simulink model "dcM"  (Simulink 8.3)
settings: Solver=ode45  StartTime=0.0  StopTime=2  FixedStep=1e-6  MaxStep=0.00001  RelTol=1e-3  AbsTol=1e-3
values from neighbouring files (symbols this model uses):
  ke = 2    [set_ga.m]
  Ra = Pcun/(Ian^2)    [Ex5i_dcMd.m]    (also in Ex6i_dcMs.m = Pcun/(In^2))
undefined symbols (not defined in the file or in its folder): B, J, Lt, period, y

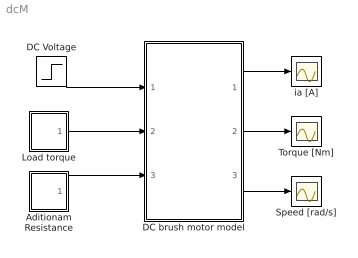
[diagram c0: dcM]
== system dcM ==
  Aditionam Resistance : Subsystem
  DC Voltage : Step  Time=0.1  After=110  SampleTime=0
  DC brush motor model : Subsystem
  Load torque : Subsystem
  Speed [rad/s] : Scope
  Torque [Nm] : Scope
  ia [A] : Scope
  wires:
  Load torque/1(out_1) -> DC brush motor model/2(Tl)
  DC brush motor model/2(Tem) -> Torque [Nm]/1
  DC brush motor model/1(Ia) -> ia [A]/1
  DC brush motor model/3(n) -> Speed [rad/s]/1
  DC Voltage/1 -> DC brush motor model/1(Va)
  Aditionam Resistance/1(out_1) -> DC brush motor model/3(Radd)

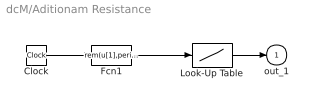
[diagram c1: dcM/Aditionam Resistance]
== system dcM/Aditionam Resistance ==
  Clock : Clock
  Fcn1 : Fcn  Expr=rem(u[1],period)
  Look-Up Table : Lookup  InputValues=t  Table=y
  out_1 : Outport
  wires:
  Fcn1/1 -> Look-Up Table/1
  Clock/1 -> Fcn1/1
  Look-Up Table/1 -> out_1/1

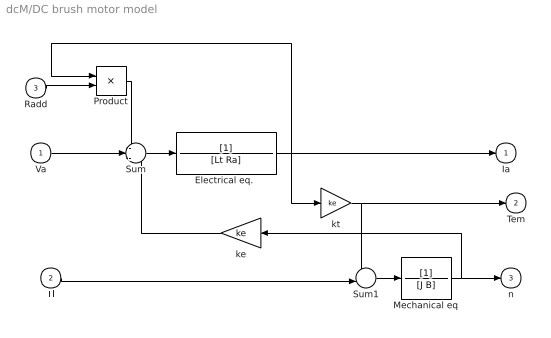
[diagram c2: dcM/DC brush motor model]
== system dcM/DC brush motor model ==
  Va : Inport
  Tl : Inport  Port=2
  Radd : Inport  Port=3
  "Electrical eq. " : TransferFcn  Denominator=[Lt Ra]
  Mechanical eq : TransferFcn  Denominator=[J B]
  Product : Product
  Sum : Sum  Inputs=-+-
  Sum1 : Sum  Inputs=+-|
  ke : Gain  Gain=ke
  kt : Gain  Gain=ke
  Ia : Outport
  Tem : Outport  Port=2
  n : Outport  Port=3
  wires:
  kt/1 -> Sum1/1, Tem/1
  "Electrical eq. "/1 -> Ia/1, kt/1, Product/1
  Sum/1 -> "Electrical eq. "/1
  Tl/1 -> Sum1/2
  Sum1/1 -> Mechanical eq/1
  Mechanical eq/1 -> n/1, ke/1
  Radd/1 -> Product/2
  Va/1 -> Sum/2
  Product/1 -> Sum/1
  ke/1 -> Sum/3

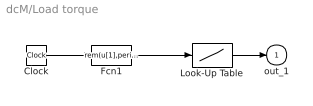
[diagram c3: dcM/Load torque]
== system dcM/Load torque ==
  Clock : Clock
  Fcn1 : Fcn  Expr=rem(u[1],period)
  Look-Up Table : Lookup  InputValues=t  Table=y
  out_1 : Outport
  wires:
  Look-Up Table/1 -> out_1/1
  Clock/1 -> Fcn1/1
  Fcn1/1 -> Look-Up Table/1
